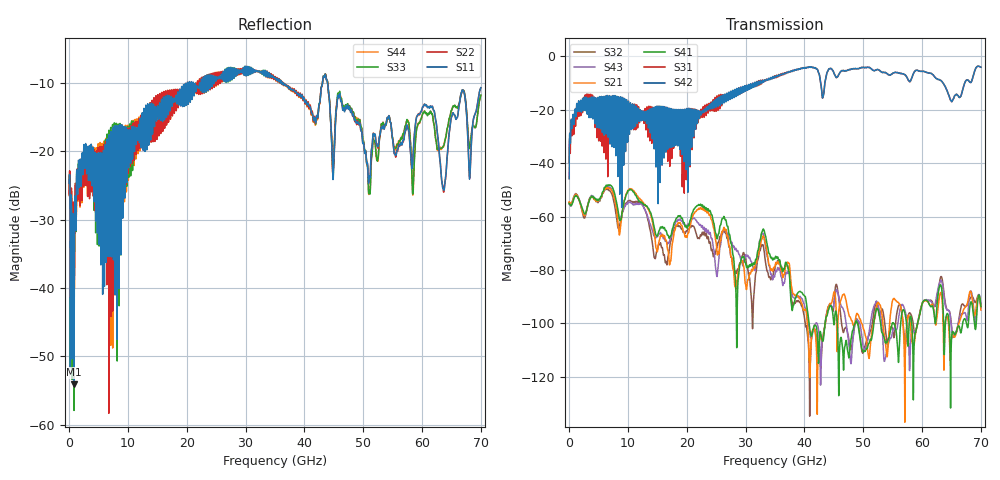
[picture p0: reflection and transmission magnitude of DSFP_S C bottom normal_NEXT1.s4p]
! AWR Design Environment (8415) Wed Jan 09 13:24:51 2019
! Document = 'DSFP_S'
! nPorts: 4, nXvals: 7001
# HZ S DB R 50
!Freq DBS11 AngS11 DBS12 AngS12 DBS13 AngS13 DBS14 AngS14
!	DBS21 AngS21 DBS22 AngS22 DBS23 AngS23 DBS24 AngS24
!	DBS31 AngS31 DBS32 AngS32 DBS33 AngS33 DBS34 AngS34
!	DBS41 AngS41 DBS42 AngS42 DBS43 AngS43 DBS44 AngS44
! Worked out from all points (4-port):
!   7000 points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, 10 MHz to 70 GHz, reference 50 ohm
!   strongest paths, dB at 10 MHz, 17.51 GHz, 35.01 GHz, 52.51 GHz, 70 GHz:
!     S42: -45.8, -28.8, -7.6, -5.0, -4.0
!     S31: -39.7, -27.3, -7.3, -4.9, -4.0
!     S41: -55.1, -65.0, -75.6, -94.9, -93.6
!     S21: -54.5, -70.6, -78.4, -92.1, -95.0
!     S43: -55.3, -65.4, -81.7, -92.7, -92.6
!     S32: -54.8, -66.4, -79.2, -93.7, -93.8
!   lowest |S11| = -54.1 dB at 850 MHz (marker M1), VSWR 1.00, Z = 50.2 + j0.0516 ohm
!   |S11| at or under -10 dB: start of sweep to 20.09 GHz; 36.44 GHz to 43.07 GHz (6.634 GHz wide, 16.7 % of centre); 43.95 GHz to end of sweep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
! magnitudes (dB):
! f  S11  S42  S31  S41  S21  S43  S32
! 10 MHz  -24.6  -45.8  -39.7  -55.1  -54.5  -55.3  -54.8
! 850 MHz  -54.1  -25.3  -26.2  -53.0  -52.5  -52.9  -52.3
! 12.22 GHz  -18.0  -23.8  -21.5  -54.6  -53.7  -55.2  -54.8
! 16.5 GHz  -14.2  -28.3  -29.2  -65.2  -68.8  -69.0  -76.8
! 22.38 GHz  -11.0  -21.5  -20.5  -55.4  -56.7  -63.2  -66.9
! 28.48 GHz  -7.9  -12.3  -12.5  -106.5  -85.4  -72.8  -81.1
! 70 GHz  -10.7  -4.0  -4.0  -93.6  -95.0  -92.6  -93.8
